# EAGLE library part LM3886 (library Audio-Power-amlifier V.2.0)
LM3886 Overture™ Audio Power Amplifier Series High-Performance 68W Audio Power Amplifier w/Mute
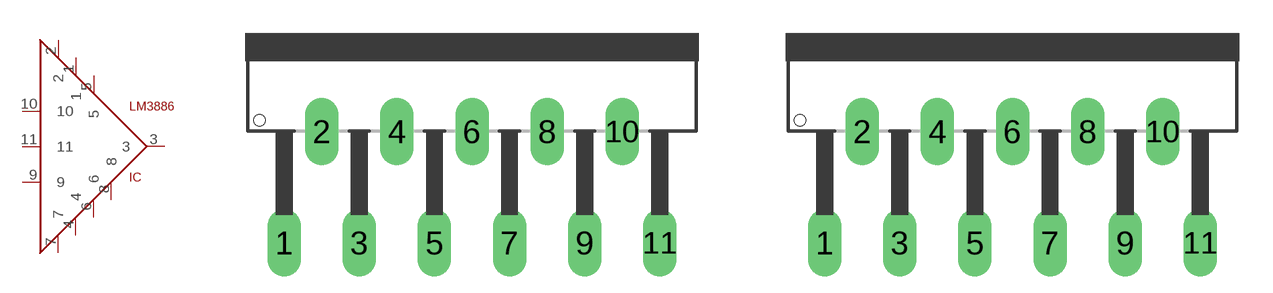
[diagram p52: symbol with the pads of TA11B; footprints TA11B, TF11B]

Designator prefix IC

## LM3886  [TA11B]
1  1  pwr
2  2  pwr
3  3  out
4  4  pwr
5  5  pwr
6  6  nc
7  7  pwr
8  8
9  9
10  10  in
11  11  nc

## LM3886TF11B  [TF11B]
Pads as for TA11B

## Footprint TA11B (pad centres in mm)
TO-220 11 lead, National Semiconductor
drill 1.016 long: 1 -8.509,-9.525; 2 -6.807,-4.47; 3 -5.105,-9.525; 4 -3.404,-4.47; 5 -1.702,-9.525; 6 0,-4.47; 7 1.702,-9.525; 8 3.404,-4.47; 9 5.105,-9.525; 10 6.807,-4.47; 11 8.509,-9.525

## Footprint TF11B (pad centres in mm)
TO-220 11 lead, National Semiconductor
drill 1.016 long: 1 -8.509,-9.525; 2 -6.807,-4.47; 3 -5.105,-9.525; 4 -3.404,-4.47; 5 -1.702,-9.525; 6 0,-4.47; 7 1.702,-9.525; 8 3.404,-4.47; 9 5.105,-9.525; 10 6.807,-4.47; 11 8.509,-9.525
